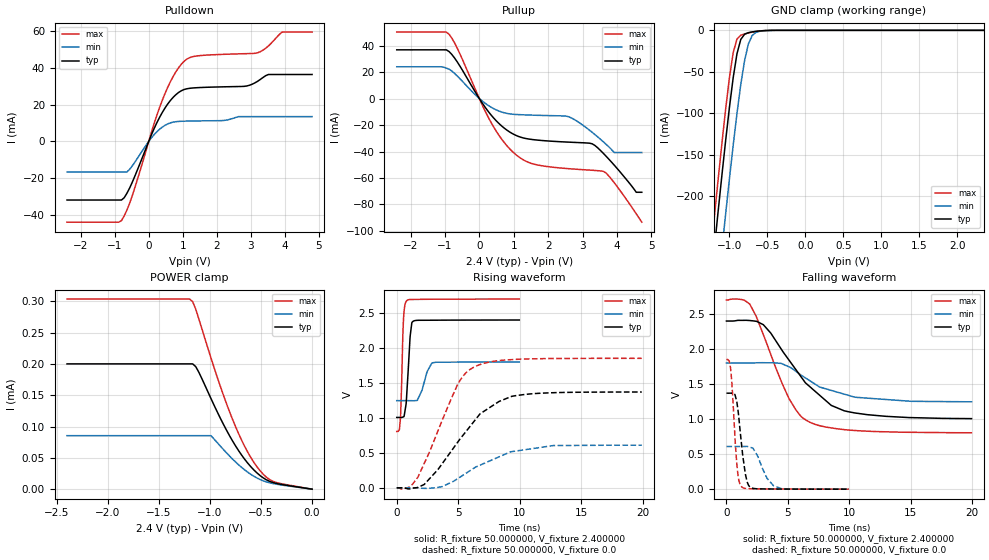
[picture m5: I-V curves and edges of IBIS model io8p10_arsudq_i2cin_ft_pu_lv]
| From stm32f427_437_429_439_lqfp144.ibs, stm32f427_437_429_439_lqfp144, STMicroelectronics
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|   Model io8p10_arsudq_i2cin_ft_pu_lv
[Model]  io8p10_arsudq_i2cin_ft_pu_lv
Model_type I/O
Polarity   Non-Inverting
Enable   Active-Low
Vinl =   0.720000V
Vinh =   1.680000V
Vmeas =  1.200000V
Cref =   40.000000pF
Rref =   100.000000M
Vref =   0.0V
C_comp   2.230300pF   2.174000pF   2.332300pF
[Temperature Range]   25.000000   0.125000k   -40.000000
[Pullup Reference]   2.400000V   1.800000V   2.700000V
[Pulldown Reference]   0.0V   0.0V   0.0V
[POWER Clamp Reference]   2.400000V   1.800000V   2.700000V
[GND Clamp Reference]   0.0V   0.0V   0.0V
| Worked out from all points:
|   slope of the pulldown table from 0 to 0.36 V, typ, clamps not added: 25 ohm
|   slope of the pullup table from 0 to 0.36 V, typ, clamps not added: 27.7 ohm
|   GND clamp passes 1 mA (typ) near -0.62 V on its own axis
|   rising waveform, R_fixture 50.000000, V_fixture 2.400000: 20-80 % time 277ps typ, 605ps min, 183ps max; typ from 1.01 V to 2.4 V
|   rising waveform, R_fixture 50.000000, V_fixture 0.0: 20-80 % time 3.71ns typ, 4.03ns min, 2.68ns max; typ from 0.001 V to 1.37 V
|   falling waveform, R_fixture 50.000000, V_fixture 2.400000: 20-80 % time 3.94ns typ, 3.97ns min, 2.73ns max; typ from 2.4 V to 1.01 V
|   falling waveform, R_fixture 50.000000, V_fixture 0.0: 20-80 % time 531ps typ, 979ps min, 385ps max; typ from 1.37 V to 0.001 V
[Pulldown]
|Voltage   I(typ)   I(min)   I(max)
-2.4V     -31.73mA   -16.51mA   -43.74mA
-800mV    -31.73mA   -16.51mA   -42.87mA
-480mV    -21.98mA   -13.17mA   -29.21mA
80mV      3.63mA     1.966mA    5.014mA
480mV     18.16mA    8.738mA    26.02mA
800mV     25.38mA    10.72mA    37.77mA
1.12V     28.53mA    11.02mA    44.6mA
2.8V      29.84mA    13.46mA    47.53mA
3.2V      32.6mA     13.46mA    48.03mA
3.52V     36.28mA    13.46mA    51.75mA
3.92V     36.28mA    13.46mA    59.24mA
4.8V      36.28mA    13.46mA    59.24mA
[Pullup]
|Voltage   I(typ)   I(min)   I(max)
-2.4V     36.81mA    24.03mA    50.22mA
-960mV    36.81mA    23mA       50.22mA
-640mV    27.63mA    17.02mA    37.96mA
320mV     -11.75mA   -6.207mA   -17.08mA
960mV     -26.47mA   -11.82mA   -40.02mA
1.52V     -30.88mA   -12.51mA   -49.05mA
2.56V     -32.88mA   -13.48mA   -52.9mA
3.28V     -34.18mA   -25.52mA   -54.17mA
3.6V      -41.3mA    -32.61mA   -54.97mA
3.92V     -50.32mA   -40.8mA    -63.62mA
4.56V     -70.8mA    -40.8mA    -87.07mA
4.72V     -70.8mA    -40.8mA    -93.4mA
[GND_clamp]
|Voltage   I(typ)   I(min)   I(max)
-2.4V     -1.424A    -1.508A    -1.393A
-1.25V    -311.2mA   -401.9mA   -273.3mA
-1.2V     -265.4mA   -356.1mA   -227.2mA
-1.15V    -220.4mA   -310.8mA   -181.9mA
-1.1V     -176.3mA   -266.2mA   -137.9mA
-1.05V    -133.8mA   -222.5mA   -95.87mA
-950mV    -57.3mA    -138.9mA   -26.98mA
-900mV    -28.27mA   -100.4mA   -10.59mA
-850mV    -11.01mA   -65.54mA   -5.958mA
-750mV    -2.834mA   -16.5mA    -3.178mA
-600mV    -750uA     -1.164mA   -738.3uA
2.35V     0A         0A         0A
[POWER_clamp]
|Voltage   I(typ)   I(min)   I(max)
-2.4V     200uA      85.39uA    303.5uA
-1.2V     200uA      85.39uA    303.5uA
-1.17V    200uA      85.39uA    299.5uA
-1.14V    195.7uA    85.39uA    287.5uA
-990mV    144.6uA    85.39uA    209.3uA
-870mV    104.1uA    63.61uA    150.8uA
-780mV    77.28uA    48.2uA     111.8uA
-660mV    47.71uA    30.75uA    68.21uA
-570mV    30.64uA    20.61uA    42.79uA
-480mV    18.19uA    13.44uA    24.07uA
-390mV    10.91uA    9.231uA    13.01uA
0V        0A         0A         0A
[Ramp]
| variable   typ   min   max
dV/dt_r  0.82195/3.70461n   0.36617/4.03289n   1.11083/2.67438n
dV/dt_f  0.83286/3.94495n   0.33240/4.02840n   1.13555/2.72505n
R_load = 50.000000
[Rising Waveform]
R_fixture= 50.000000
V_fixture= 2.400000
V_fixture_min= 1.800000
V_fixture_max= 2.700000
|time   V(typ)   V(min)   V(max)
0s        1.007V     1.247V     805.7mV
200.2ps   1.007V     1.247V     826.8mV
300.3ps   1.007V     1.247V     990.9mV
560.6ps   1.017V     1.247V     2.445V
820.8ps   1.356V     1.247V     2.677V
1.101ns   2.184V     1.247V     2.693V
1.341ns   2.383V     1.246V     2.694V
1.682ns   2.395V     1.253V     2.695V
2.883ns   2.397V     1.788V     2.697V
9.97ns    2.4V       1.8V       2.699V
[Rising Waveform]
R_fixture= 50.000000
V_fixture= 0.0
V_fixture_min= 0.0
V_fixture_max= 0.0
|time   V(typ)   V(min)   V(max)
0s        1.049mV    906.3uV    1.472mV
1.121ns   -12.04mV   969.1uV    18.34mV
1.722ns   8.574mV    -206.6uV   153mV
3.323ns   256.5mV    6.122mV    802.4mV
4.925ns   644.9mV    128.6mV    1.467V
6.206ns   932.5mV    274.3mV    1.719V
6.807ns   1.062V     327.3mV    1.765V
9.369ns   1.31V      518.9mV    1.834V
12.73ns   1.361V     605mV      1.849V
19.94ns   1.371V     610.2mV    1.852V
[Falling Waveform]
R_fixture= 50.000000
V_fixture= 2.400000
V_fixture_min= 1.800000
V_fixture_max= 2.700000
|time   V(typ)   V(min)   V(max)
0s        2.4V       1.8V       2.699V
1.121ns   2.41V      1.8V       2.71V
1.882ns   2.407V     1.801V     2.644V
3.003ns   2.348V     1.805V     2.205V
5.085ns   1.844V     1.747V     1.296V
6.046ns   1.611V     1.633V     1.042V
6.767ns   1.466V     1.55V      957.4mV
8.529ns   1.196V     1.41V      875.2mV
9.85ns    1.108V     1.343V     845.9mV
19.94ns   1.007V     1.247V     805.7mV
[Falling Waveform]
R_fixture= 50.000000
V_fixture= 0.0
V_fixture_min= 0.0
V_fixture_max= 0.0
|time   V(typ)   V(min)   V(max)
0s        1.371V     610.2mV    1.852V
340.3ps   1.371V     610.2mV    1.719V
440.4ps   1.371V     610.2mV    1.521V
700.7ps   1.344V     610.1mV    721.3mV
940.9ps   1.123V     609.9mV    201mV
1.221ns   652.6mV    609.7mV    37.95mV
1.682ns   105.7mV    611.3mV    8.237mV
2.042ns   19.33mV    591.8mV    6.362mV
3.844ns   3.103mV    48.82mV    2.614mV
9.97ns    1.049mV    906.3uV    1.472mV
